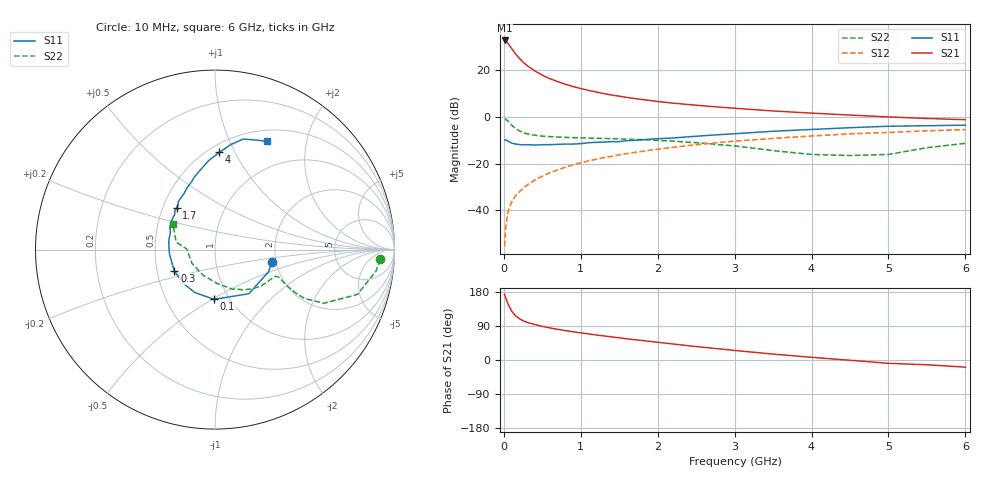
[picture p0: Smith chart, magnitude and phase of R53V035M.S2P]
! SIEMENS Small Signal Semiconductors
! BFR183
! Si NPN RF Bipolar Junction Transistor in SOT23
! VCE = 3 V  IC = 35 mA
! Common Emitter S-Parameters:  May  1996
# GHz  S  MA  R  50
!  f  S11  S21  S12  S22
! GHz  MAG  ANG  MAG  ANG  MAG  ANG  MAG  ANG
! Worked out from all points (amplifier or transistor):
!   36 points, 10 MHz to 6 GHz, reference 50 ohm
!   highest |S21| = 32.9 dB at 10 MHz (marker M1)
!   |S21| within 3 dB of that: start of sweep to 91.47 MHz
!   unconditionally stable (mu >= 1): 372.6 MHz to 2.367 GHz
!   at 250 MHz: K = 0.93, MSG = 27.1 dB, |S12| = -30.6 dB
!   at 1.4 GHz: K = 1.06, MAG = 11.7 dB, |S12| = -16.8 dB
!   at 6 GHz: K = 0.91, MSG = 2.1 dB, |S12| = -5.4 dB
!   S11 on the Smith chart (normalised r, x): 10 MHz: 1.90, -0.28; 100 MHz: 0.85, -0.51; 300 MHz: 0.62, -0.16; 1.7 GHz: 0.59, +0.31; 4 GHz: 0.57, +0.87; 6 GHz: 0.64, +1.39
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0.01  0.3232 -11.9  43.99 173.2  0.0017 79.8  0.922 -3.4
0.02  0.3235 -22.4  43.33 166.6  0.0037 80.4  0.905 -7.6
0.05  0.3096 -52.6  39.01 149.7  0.0088 74.8  0.8319 -17.5
0.1  0.2773 -91.1  29.73 129.7  0.0149 72.0  0.6767 -26.2
0.15  0.2643 -115.4  22.86 117.1  0.0202 70.5  0.5701 -28.6
0.2  0.2575 -130.9  18.3 109.3  0.0248 72.3  0.5063 -28.2
0.25  0.2531 -143.5  15.05 103.7  0.0296 72.3  0.4645 -27.2
0.3  0.2561 -152.2  12.8 99.5  0.0345 73.6  0.4385 -26.3
0.4  0.2509 -164.6  9.822 93.7  0.0443 74.1  0.408 -24.6
0.5  0.2548 -174.3  7.905 88.7  0.054 74.5  0.3901 -23.5
0.6  0.2563 178.5  6.655 84.6  0.0641 74.8  0.38 -23.4
0.8  0.2634 167.3  5.054 77.6  0.0841 73.2  0.3668 -24.1
0.9  0.2636 161.7  4.508 74.5  0.0945 73.0  0.3617 -24.7
1.1  0.2811 153.6  3.741 68.9  0.1144 71.2  0.3549 -27.3
1.4  0.2961 141.3  2.973 61.0  0.1438 68.3  0.3452 -31.1
1.7  0.3164 132.3  2.494 53.6  0.1745 65.1  0.3313 -35.8
2.2  0.3556 119.2  1.988 42.2  0.2248 59.3  0.3052 -45.6
3.5  0.4963 94.2  1.352 15.6  0.3482 42.0  0.1907 -85.5
4  0.5423 87.4  1.215 7.1  0.3922 35.8  0.1577 -114.7
4.5  0.5915 81.5  1.103 -0.7  0.4362 28.9  0.1497 -149.0
5.5  0.6521 69.3  0.933 -12.6  0.5066 16.8  0.2205 169.1
6  0.6699 64.2  0.877 -18.9  0.5391 9.1  0.2734 148.8
